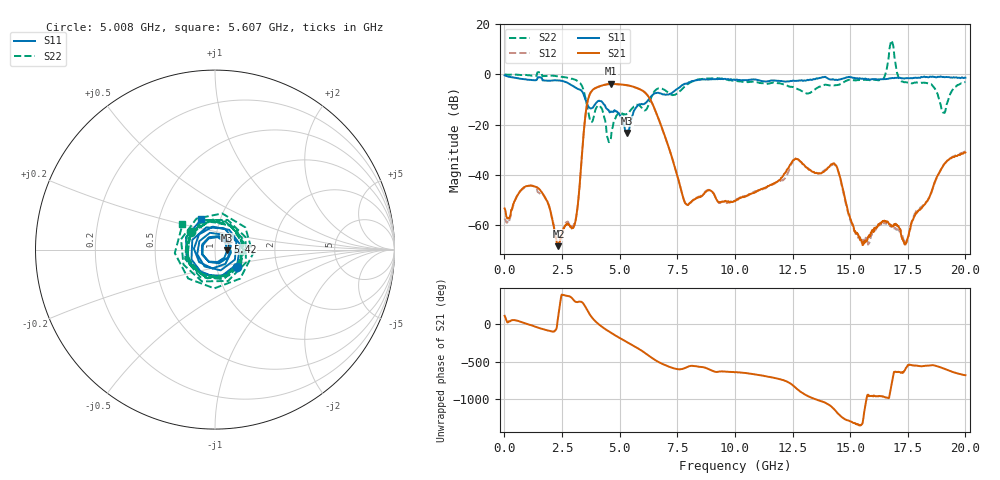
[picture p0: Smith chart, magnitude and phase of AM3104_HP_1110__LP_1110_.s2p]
!Created with skrf (http://scikit-rf.org).
# Hz S RI R 50.0
!freq ReS11 ImS11 ReS21 ImS21 ReS12 ImS12 ReS22 ImS22
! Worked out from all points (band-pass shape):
!   1601 points, 10 MHz to 20 GHz, reference 50 ohm
!   highest |S21| = -3.75 dB at 4.633 GHz (marker M1); lowest = -68.3 dB at 2.346 GHz (marker M2)
!   |S21| within 3 dB of the highest: 3.779 GHz to 6.041 GHz (2.262 GHz wide, 46.1 % of centre)
!   lowest |S11| = -23.2 dB at 5.32 GHz (marker M3), VSWR 1.15, Z = 57.4 - j0.406 ohm
!   |S11| at or under -10 dB: 3.517 GHz to 6.259 GHz (2.742 GHz wide, 56.1 % of centre)
!   |S22| runs from -26.9 to 13.5 dB; largest |S21 - S12| = 0.075
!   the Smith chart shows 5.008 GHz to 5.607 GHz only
!   S11 on the Smith chart (normalised r, x): 5.008 GHz: 1.25, -0.25; 5.42 GHz: 1.15, +0.10; 5.607 GHz: 0.81, +0.28
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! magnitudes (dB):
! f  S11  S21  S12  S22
! 10 MHz  -0.4  -53.3  -57.3  0.0
! 1.259 GHz  -2.3  -44.5  -44.4  -0.5
! 2.346 GHz  -2.4  -68.3  -68.2  -0.8
! 3.046 GHz  -5.0  -59.8  -59.5  -2.0
! 3.346 GHz  -6.5  -34.4  -34.6  -4.2
! 3.696 GHz  -13.3  -8.1  -8.1  -17.3
! 4.145 GHz  -10.6  -4.7  -4.7  -12.7
! 4.633 GHz  -14.8  -3.7  -3.9  -24.3
! 5.008 GHz  -16.1  -4.0  -4.0  -15.5
! 5.32 GHz  -23.2  -4.3  -4.3  -15.8
! 5.42 GHz  -21.6  -4.5  -4.5  -14.9
! 5.607 GHz  -14.7  -4.9  -5.0  -12.8
! 6.682 GHz  -7.3  -17.5  -17.5  -5.5
! 7.881 GHz  -3.7  -51.5  -51.4  -4.4
! 10.01 GHz  -2.2  -50.5  -50.0  -2.7
! 13.34 GHz  -2.2  -38.6  -38.6  -6.9
! 14.37 GHz  -2.1  -36.1  -36.3  -4.3
! 15.54 GHz  -1.6  -67.9  -67.0  -2.2
! 16.68 GHz  -1.6  -59.4  -59.8  7.2
! 17.43 GHz  -1.5  -66.9  -66.9  -3.1
! 19.05 GHz  -1.0  -36.1  -36.0  -15.2
! 20 GHz  -1.3  -31.0  -30.7  -3.0
